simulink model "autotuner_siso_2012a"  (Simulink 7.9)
settings: Solver=ode3  StartTime=0.0  StopTime=simopt.Tf  FixedStep=simopt.h  RelTol=1e-3
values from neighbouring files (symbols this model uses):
  params = []    [setParams.m]
  simopt = []    [setParams.m]
libraries: simulink x1

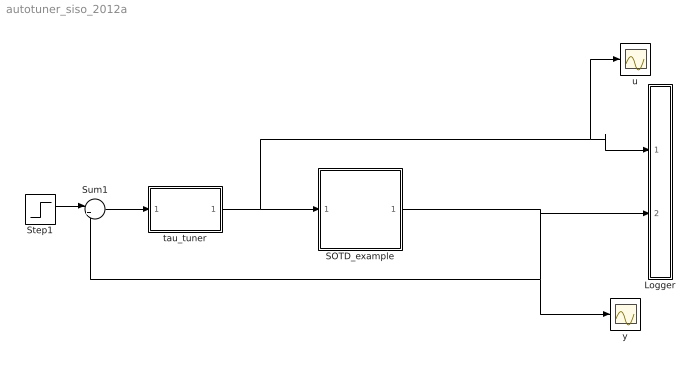
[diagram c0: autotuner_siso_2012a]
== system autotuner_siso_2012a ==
  Logger : Subsystem
  SOTD_example : Subsystem
  Step1 : Step  Time=0  After=0  SampleTime=simopt.h
  Sum1 : Sum  Inputs=|+-
  tau_tuner : Subsystem
  u : Scope
  y : Scope
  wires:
  tau_tuner/1(u) -> u/1, Logger/1(u1), SOTD_example/1(u)
  Step1/1 -> Sum1/1
  Sum1/1 -> tau_tuner/1(e)
  SOTD_example/1(y) -> Logger/2(y1), y/1, Sum1/2

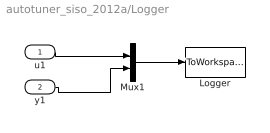
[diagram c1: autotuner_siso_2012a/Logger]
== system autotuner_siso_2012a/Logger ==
  u1 : Inport  SampleTime=simopt.h
  y1 : Inport  Port=2  SampleTime=simopt.h
  Logger : ToWorkspace  VariableName=simout  SampleTime=simopt.h  SaveFormat=Structure With Time
  Mux1 : Mux  Inputs=2
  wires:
  u1/1 -> Mux1/1
  y1/1 -> Mux1/2
  Mux1/1 -> Logger/1

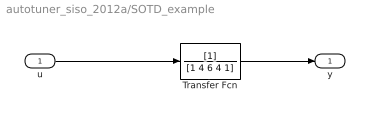
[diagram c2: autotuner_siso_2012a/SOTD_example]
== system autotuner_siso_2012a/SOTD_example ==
  u : Inport  SampleTime=simopt.h
  Transfer Fcn : TransferFcn  Denominator=[1 4 6 4 1]
  y : Outport  SampleTime=simopt.h
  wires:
  u/1 -> Transfer Fcn/1
  Transfer Fcn/1 -> y/1

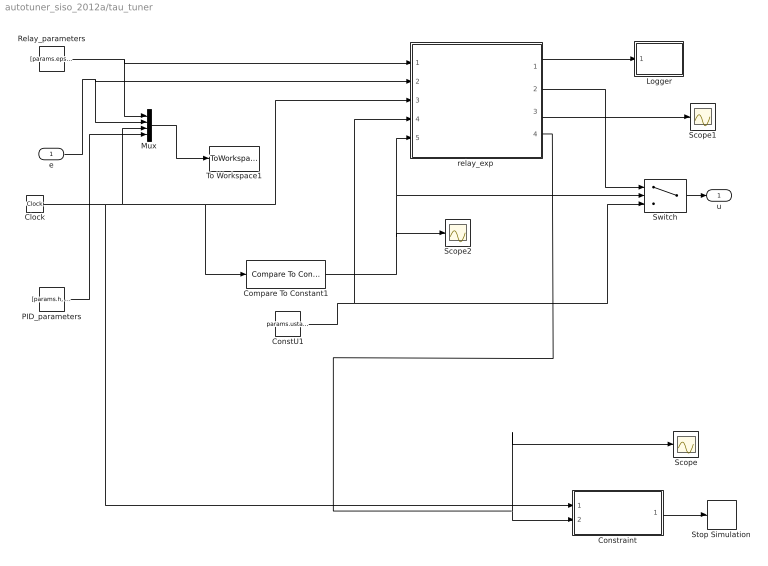
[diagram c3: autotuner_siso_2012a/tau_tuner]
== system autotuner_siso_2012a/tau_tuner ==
  e : Inport  SampleTime=simopt.h
  Clock : Clock
  Compare To Constant1 : simulink/Logic and Bit Operations/Compare To Constant  relop=>=  const=params.expStartTime  OutDataTypeStr=boolean
  ConstU1 : Constant  Value=params.ustart  SampleTime=simopt.h
  Constraint : MATLAB Function  TreatAsAtomicUnit=on
  Logger : Subsystem
  Mux : Mux
  PID_parameters : Constant  Value=[params.h, params.equi]  SampleTime=simopt.h
  Relay_parameters : Constant  Value=[params.eps, params.asym, params.h, 2,12,1, params.uon,params.hyst,params.noiseMeasureTime, 0]  SampleTime=simopt.h
  Scope : Scope
  Scope1 : Scope
  Scope2 : Scope
  Stop Simulation : Stop
  Switch : Switch  Criteria=u2 ~= 0
  To Workspace1 : ToWorkspace  VariableName=result1  SampleTime=-1  SaveFormat=Timeseries
  "relay_exp " : MATLAB Function  TreatAsAtomicUnit=on
  u : Outport  SampleTime=simopt.h
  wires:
  Constraint/1(stop) -> Stop Simulation/1
  "relay_exp "/1(result) -> Logger/1(result)
  "relay_exp "/3(PID_param) -> Scope1/1
  Clock/1 -> Constraint/1(time), Mux/3, "relay_exp "/3(t), Compare To Constant1/1
  "relay_exp "/4(done) -> Scope/1, Constraint/2(done)
  ConstU1/1 -> Switch/3, "relay_exp "/4(u_ref)
  Compare To Constant1/1 -> Switch/2, "relay_exp "/5(run_exp), Scope2/1
  "relay_exp "/2(u) -> Switch/1
  PID_parameters/1 -> Mux/4
  Relay_parameters/1 -> Mux/1, "relay_exp "/1(relay_par)
  e/1 -> Mux/2, "relay_exp "/2(e)
  Switch/1 -> u/1
  Mux/1 -> To Workspace1/1

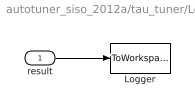
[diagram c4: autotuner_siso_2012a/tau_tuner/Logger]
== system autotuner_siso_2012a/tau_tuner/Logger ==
  result : Inport  SampleTime=simopt.h
  Logger : ToWorkspace  VariableName=result  SampleTime=simopt.h  SaveFormat=Structure With Time
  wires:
  result/1 -> Logger/1

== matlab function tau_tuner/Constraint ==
%function stop = Constraint(tstop, time, done)
function stop = Constraint(time, done)
%#codegen
persistent tstopp
if isempty(tstopp)
    tstopp = 10000;
end
if done == 1
    tstopp = time;
end
if time > tstopp; %+params.timeAfterExp;
    stop = 1;
else
    stop = 0;
end

== matlab function tau_tuner/relay_exp
 ==
function [result, u, PID_param, done]= relay_exp(relay_par, e,t, u_ref, run_exp)


%%%%%%%%%% Definitions and default values %%%%%%%%%%%%%%
y = -e;
% Relay parameters, values from workspace.
persistent d1 d2 u_on u_off h
epsilon = relay_par(1);
gamma = relay_par(2); 
t_sample = relay_par(3);
low_limit_f = relay_par(4);
upp_limit_f = relay_par(5);
bigYup = relay_par(6);
relayMaxDev = relay_par(7);
def_h = relay_par(8);
noiseMeasureTime = relay_par(9);
fixAmp = relay_par(10);

persistent yref uref resultvec
if isempty(d2)
    h=def_h;
    % These values are assigned to their values later in the code, but in an if-statement
    % so the program doesn't understand that they will always be assigned. 
    d1 = gamma;
    d2 = 1;
    u_on =  d1;
    u_off = -d2;
    uref = 0;
    yref = y;
    resultvec = zeros(22,1);
end

% Creating arrays for data logging
maxlength = 1000000;
persistent uvec yvec tvec 
if isempty(uvec)
    uvec = zeros(1,maxlength);
    yvec = zeros(1,maxlength);
    tvec = zeros(1,maxlength);
end

persistent sample
if isempty(sample)
    sample = 0;
end

persistent startup Ksign startup_switch amp_changed
if isempty(Ksign)
    Ksign = 1; % Is found and assigned during the startup phase
    startup_switch = 0; 
    amp_changed = 0;
end

persistent param 
if isempty(param)
    param = [1, 10, 0]; % Should be an input somehow if an existing PID controller is used first
end
PID_param = param; % Not allowed to have a persistent variable as output so had to do like this
done = 0;
finished = false;

% To handle switches
persistent switching_times switch_index last_switch_sample
if isempty(switching_times)
    switching_times = zeros(1,100); % Larger than necessary
    switch_index = 1;
    last_switch_sample = 1;
end

%%%%%%%%% Startup  params %%%%%%%%%%%
persistent a b c ttf exp_t yh yl measureNoise first
if isempty(startup)
    uvec(1) = uref;
    yvec(1) = yref;
    tvec(1) = 0;
    ttf = 5/t_sample; % Want to run the exponential growth for a certain time, not a number of samples. According to Tore about 3-5s 
    b = 40;
    c = relayMaxDev/(b-1);
    a = uvec(1)-c;
    measureNoise = 1;
    startup = 0;
    yh = 0;
    yl = 0;
    first = true;
end
%%%%%%%%%%%%%%%%%%%%%%%%%%%%%%%%%%%%%%%%%%%%%%%

result = resultvec;
if run_exp == 0
    done = 0;
    u = 0;
    PID_param = param;
    return
end
if fixAmp == 1
   d1 = upp_limit_f;
   d2 = low_limit_f;
end
%%%%%%%%%%%%% Program running %%%%%%%%%%%%%%%%%
sample = sample+1;
if sample > 1
  yvec(sample-1) = y; % store inputs
  tvec(sample) = t;
end

%%%%%%%%% Startup %%%%%%%%%%%%
if measureNoise == 1
    if first 
        uref = u_ref;
        yref = y;
        first = false;
        yh = yref;
        yl = yref;
    end
    u = uref;
    if sample < noiseMeasureTime/t_sample
        yh = max(yh,y);
        yl = min(yl,y);
    else
        resultvec(13) = yh;
        resultvec(14) = yl;
        noise = (yh-yl)/2;
        yref = (yh+yl)/2;
        resultvec(15) = yref;
        resultvec(16) = uref;
        h = max(2*noise, def_h);
        resultvec(12) = h;
        measureNoise = 0;
        startup = 1;
    end
elseif startup == 1
    exp_t = sample-noiseMeasureTime/t_sample; % this should be zero the first sample
    a = uref-c;
        u = a+c*b^(exp_t/ttf);
        if u > relayMaxDev+uref
            u = relayMaxDev+uref;
        end
        if exp_t > 1
            ydev = y-yref; 
            if abs(ydev) > h % when reached outside hysteresis, stop and decide Ksign
                Ksign = ydev/abs(ydev)
                if bigYup == 1
                    d1 = min(relayMaxDev, gamma*abs(u-uref));
                    d2 = d1/gamma;
                else
                    d2 = min(relayMaxDev, gamma*abs(u-uref));
                    d1 = d2/gamma;
                end
                startup = 0;
                startup_switch = 1; % To not immediately change the new amplitude.
            elseif exp_t > ttf
                u = uref+relayMaxDev;
            end
        end
elseif done == 0
    %%%%%% Update amplitudes %%%%%%%
    u_on = uref+Ksign*d1;
    u_off = uref-Ksign*d2;
    %%%%%% Calculate new u %%%%%%%%%
    u = rel_func(y,uvec(sample-1),u_on, u_off,yref,h);
else 
    u = 0; % If the experiment aren't running no control signal should be calculated here
    % This script shouldn't be running in those cases but somehow it seems
    % to do.
end
%%%% store data %%%%%%
uvec(sample) = u;

%%%%%%% At switching points %%%%%%%
if sample>1 && (uvec(sample)-uref)*(uvec(sample-1)-uref) < 0
    switching_times(switch_index) = tvec(sample);
    low_limit = low_limit_f*h;
    upp_limit = upp_limit_f*h;
    ratio = check_amplitudes(yvec(last_switch_sample:sample-1)-yref, upp_limit, low_limit, gamma);
    if fixAmp == 1
        ratio = 1;
    end
    if amp_changed == 1 % To not change two consecutive half periods...
        ratio = 1;
        amp_changed = 0;
    end
    if (ratio > 1.01 || ratio < 0.99) && startup_switch ~= 1 
        if max(d1,d2)*ratio > relayMaxDev
            if max(d1,d2) == relayMaxDev
                ratio_forced = 1
                %ratio = 1;
            else
                ratio = relayMaxDev/max(d1,d2);
                d1 = d1*ratio;
                d2 = d2*ratio;
                switch_index = 0; % to reset convergence checks if changed amplitude.
                amp_changed = 1;
            end
            
       else
            d1 = d1*ratio;
            d2 = d2*ratio;
            switch_index = 0; % To reset convergence checks if changed amplitude.
            amp_changed = 1;
       end
       if uvec(sample) == u_on
           u = uref+Ksign*d1;
       elseif uvec(sample) == u_off
           u = uref-Ksign*d2;
       else
           error = 1
       end
       uvec(sample) = u;
    end
    startup_switch = 0;
    if switch_index > 3
        tp = switching_times(switch_index)-switching_times(switch_index-2);
        tp_old = switching_times(switch_index-1)-switching_times(switch_index-3);
        resultvec(19) = tp;
        resultvec(20) = tp_old;
        if abs(tp-tp_old)<tp_old*epsilon
            finished = true;
            tstop = tvec(sample);
            resultvec(17) = tstop;
        end
    end
    last_switch_sample = sample;
    switch_index = switch_index+1;
end


% Checks if converged, in that case collect info and call a method that
% calculates a model and PI/PID parameters
if finished == true
    tsim = tvec(1:sample);
    usim = uvec(1:sample)-uref;
    ysim = yvec(1:sample)-yref;
        u1 = usim(1:end-1);
        u2 = usim(2:end);
        switches = find(u1.*u2<0);
        yp = ysim(switches(end-2):switches(end));
        up = usim(switches(end-2):switches(end));
        tp = tsim(switches(end-2):switches(end));
        y_int = trapz(tp,yp);
        u_int = trapz(tp,up);
        resultvec(21) = y_int;
        resultvec(22) = u_int;
    [ton toff] = calc_ton_toff(usim, switching_times(1:switch_index-1), u_on-uref);
    resultvec(8) = ton;
    resultvec(9) = toff;
    %%%%% Calulating tau %%%%%
    rho = max(ton, toff)/min(ton, toff);
    tau = min(1, max((gamma-rho)/((gamma-1)*(0.35*rho+0.65)),0)) %Min&max if something strange would occur.
    resultvec(1) = tau;
  
    if tau > 0.1 % this condition needs to be considered more closely
        [K,T,L] = calc_FOTD_params(u_int,y_int,d1,d2,h,ton,toff,tau);
        if tau > 0.6
           [Kc, Ti, Td] = calc_AMIGO_PI(K,T,L);
        else
            [Kc, Ti, Td] = calc_AMIGO_PID(K,T,L);
        end
        resultvec(2) = K;
        resultvec(3) = T;
        resultvec(4) = L;
        resultvec(5) = Kc;
        resultvec(6) = Ti;
        resultvec(7) = Td;
    else
        [kv, L] = calc_integrating_params(y_int, u_on-uref, u_off-uref, ton, toff, h);
        %[Kc, Ti, Td] = calc_AMIGO_int_PI(kv, L);
        [Kc, Ti, Td] = calc_AMIGO_int_PID(kv, L); % Which one do I want?
        resultvec(2) = kv;
        resultvec(3) = -1;
        resultvec(4) = L;
        resultvec(5) = Kc;
        resultvec(6) = Ti;
        resultvec(7) = Td;
    end
    done = 1;
    param = [Kc, Ti, Td];
    resultvec(10) = d1;
    resultvec(11) = d2;
    resultvec(18) = done;
    resultvec
end
end


% ---------------------------------
 function ratio = check_amplitudes(y, upper_limit, lower_limit, gamma)
        % Is checked at every switching point and sends in y = y_vec-yref
        % for the entire half period. No point to check at other time
        % instances!
        ratio1 = max(abs(y))/upper_limit; % Top value deviates too much if > 1
        ratio2 = max(abs(y))/lower_limit; % Top value too close to hysteresis limit if < 1.
     
        if ratio1 > 1
            ratio = (upper_limit+lower_limit*gamma)/(2*max(abs(y))); 
        elseif ratio2 < 1
            ratio = (lower_limit+upper_limit/gamma)/(2*max(abs(y)));
        else
            ratio =1;
        end
    end
%---------------------------------------

function u = rel_func(y,uold,uon,uoff,yref,h)
  if y <= yref-h
    u = uon;
  elseif y < yref+h && y > yref-h
    u = uold;
  else u = uoff;
  end
end

% --------------------------------
function [ton, toff] = calc_ton_toff(u, switching_times, u_on)

if u(end-1) == u_on
    ton = switching_times(end)-switching_times(end-1);
    toff = switching_times(end-1)-switching_times(end-2);
else
    toff = switching_times(end)-switching_times(end-1);
    ton = switching_times(end-1)-switching_times(end-2);
end
end

% ---------------------------------------------------

function [kstart tstart lstart] = calc_FOTD_params(u_int,y_int,d1,d2,h, ton, toff, tau)
kstart=y_int/u_int;
LdivT = tau/(1-tau);
% Equations from commit 2015-02-10
u_int
y_int
d1
d2
h
ton
toff
tau
tstart1 = ton/log((h/abs(kstart)-d2+exp(LdivT)*(d1+d2))/(d1-h/abs(kstart)));
tstart2 = toff/log((h/abs(kstart)-d1+exp(LdivT)*(d1+d2))/(d2-h/abs(kstart)));
tstart = (tstart1+tstart2)/2;
lstart = tstart*LdivT;
end

% --------------------------------------------

function [K, Ti, Td] = calc_AMIGO_PI(Kp,T,L)
K = 0.15/Kp+(0.35-L*T/(L+T)^2)*T/(Kp*L);
Ti = 0.35*L+13*L*T^2/(T^2+12*L*T+7*L^2);
Td = 0;
end

function [K, Ti, Td] = calc_AMIGO_PID(Kp,T,L)
K = (0.2*L+0.45*T)/(Kp*L);
Ti = (0.4*L+0.8*T)/(L+0.1*T)*L;
Td = 0.5*L*T/(0.3*L+T);
end

% --------------------------------------------
function [kv, L] = calc_integrating_params(y_int, uon, uoff, ton, toff, h)
%Equations from commit 2015-02-10
y_int
uon
uoff
ton
toff
h

kv = 2*y_int/(ton*toff*(uon+uoff))+2*h/(uon*ton);
L = (uon*ton-2*h/kv)/(uon-uoff);
if L < 0
    L = 1e-3;
end
end

% -------------------------------------------
function [K, Ti, Td] = calc_AMIGO_int_PI(Kv, L)
K = 0.35/(Kv*L);
Ti = 13.4*L;
Td = 0;
end

function [K, Ti, Td] = calc_AMIGO_int_PID(Kv, L)
K = 0.45/(Kv*L);
Ti = 8*L;
Td = 0.5*L;
end
